PROGRAM PRG_Recipe_OtherHMI	(*第三方触摸屏, 参数保存, 配方功能*)
VAR
	fbRecipeOtherHMI		: FB_Recipe_OtherHMI;
	eFileType			: E_FileType :=eFileType_BIN;
END_VAR


(*测试*)
VAR
	nErrorCounter			: INT;
	nDoneCounter			: INT;
END_VAR

;
fbRecipeOtherHMI(
	bRunOnCeDevice		:= FALSE,					(* TRUE--CE系统, FALSE--非CE系统*)
	sgFilePath			:= ,						(* 文件路径, 默认是 \Data\Recipe\' *)
	eFileType			:= eFileType,						(* 文件类型, 默认是XML, 只支持 eFileType_XML 和 eFileType_BIN 两种类型 *)
	pRecData			:= ADR(sRecData),			(* 配方参数首地址 *)
	pBakData			:= ADR(_sRecData),			(* 配方备份的首地址, 保存上一次的参数值, 用来比较参数是否有变化 *)
	nRecSize			:= SIZEOF(sRecData),		(* 配方总字节数 *)
	tAutoSaveRec		:= T#10S,					(* 参数变化后, 延时保存(写文件) *)
	H_RecipeLoad		:= H_RecipeLoad,			(* 第三方触摸屏上的 读取配方 按钮 *)
	H_RecipeSave		:= H_RecipeSave,			(* 第三方触摸屏上的 保存配方 按钮 *)
	H_RecipeSaveAs		:= H_RecipeSaveAs,			(* 第三方触摸屏上的 另存配方 按钮 *)
	H_SetRecipeNum		:= H_SetRecipeNum,			(* 第三方触摸屏上的 读写配方号 *)
	H_RecipeName		:= H_RecipeName,			(* 第三方触摸屏上的 配方名(输入输出接口) *)
	H_CurRecipeNum		=> H_CurRecipeNum,			(* 当前配方号 *)
	H_CurRecName		=> H_CurRecName,			(* 当前配方名 *)
	H_RecipeInitialDone	=> H_RecipeInitialDone,		(* 初始化完成 *)
	H_RecipeDone		=> H_RecipeDone,			(* 读写完成 *)
	H_RecipeBusy		=> H_RecipeBusy,			(* 读写中 *)
	H_RecipeError		=> H_RecipeError,			(* 读写失败 *)
	H_RecipeLoading		=> H_RecipeLoading,			(* 读取配方中 *)
	H_RecipeSaving		=> H_RecipeSaving,			(* 保存配方中 *)
	H_NewRecipeSaving	=> H_NewRecipeSaving,		(* 另存配方中 *)
	H_CurDataAutoSaving	=> H_CurDataAutoSaving);	(* 自动保存中 *)


(*测试*)
IF H_RecipeError THEN
	nErrorCounter := nErrorCounter + 1;
END_IF
IF H_RecipeDone THEN
	nDoneCounter := nDoneCounter + 1;
END_IF

END_PROGRAM
